FUNCTION_BLOCK FB43
TITLE =Get Analog Input
//*****************************************************************************
//* maxon motor ag
//* R&D
//* all rights reserved
//*****************************************************************************
//* Summary:  Read analog input value
//*
//* Remarks:
//*
//* Created under: STEP7 REV5.2+SP1
//*****************************************************************************
//* History:
//* 19.05.2004 | INA   first release
//*
//*
//*****************************************************************************
//

AUTHOR:INA
FAMILY:I_O_Mode
NAME:GetAnIn
VERSION:00.01


VAR_INPUT

Read : BOOL //A rising edge start the command

  NodeID : BYTE //Adress of the maxon device

  Number : DWORD //Number of the analog input

END_VAR
VAR_OUTPUT
  Done : BOOL //Data valid flag is TRUE if data were available

  Err : BOOL //Error flag is TRUE if an Error has occured, see ErrNo for more details

  ErrNo : DINT //Contains detailed error information

  AnalogInput : WORD //State of the analog input

END_VAR
VAR
  xEdgeMerker : BOOL //Edge Merker

  xEdgeFlag : BOOL //Edge Flag

  xStep : INT
END_VAR

BEGIN

NETWORK
TITLE = Activate the service function
//

// SDO Read "Get Analog Input"

       U    #Read
       FP   #xEdgeFlag                   // recognize a positiv edge of the Read signal
       =    #xEdgeMerker                 // and set the xEdgeMerker for one cycle to true

       L    #xStep
       L    0
       ==I
       U    #xEdgeMerker
       SPB  nstp                         // iStep = 1 -> fnc1

       L    #xStep                       // jump list
       SPL  List
       SPA  rdef
       SPA  fnc1
       SPA  fncE
List  :SPA  rdef

rdef  :NOP  0
       R    #Done                        // reset Done
       R    #Err                         // reset Error
       L    0
       T    #xStep                       // iStep = 0
       SPA  end

fnc1  :NOP  0
       CALL FC1
         NodeID:=#NodeID
         Index:=DW#16#0000207C
         SubIndex:=#Number
         RET_VAL:=#Done
         Err:=#Err
         ErrNo:=#ErrNo

       L    DB219.DBW10
       T    #AnalogInput

fncE  :NOP  0
       L    0
       T    #xStep
       SPA  end

nstp  :NOP  0
       L    #xStep
       INC            1
       T    #xStep

end   :NOP  0
END_FUNCTION_BLOCK
